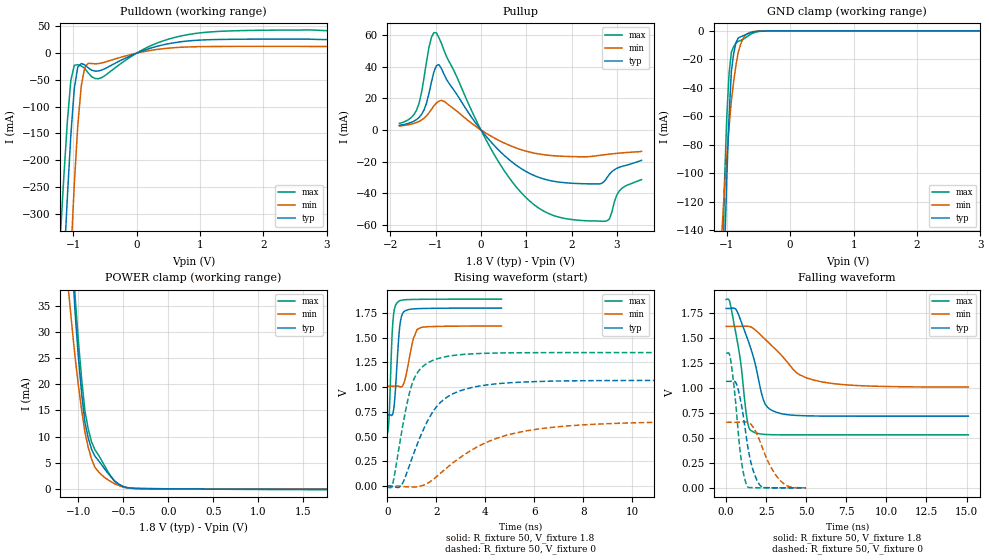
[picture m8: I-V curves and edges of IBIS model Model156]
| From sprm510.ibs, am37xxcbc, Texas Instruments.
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| Model based on original model for DSIPHY_WIO_ADDON_GPIOWRAPPER
|   Sub model FBPB_HS01L10_PU1_1P8
[model]   Model156
|[Input Load]   PU
|[Output Drive] SC01LB10
|Voltage   1.8V
|Mode   I/O
Model_type   I/O
Polarity   Non-Inverting
Enable   Active-Low
Vinl =  0.63
Vinh =  1.17
Cref =  15pF
Rref =  100.0000M
Vref =  0V
Vmeas =  0.9
C_comp   1.429432p   1.270657p   1.602015p
[Model Spec]
Vinl   0.63   0.567   0.6615
Vinh   1.17   1.053   1.2285
[Temperature Range]   25   125   -40
[Voltage Range]   1.8   1.62   1.89
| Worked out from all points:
|   slope of the pulldown table from 0 to 0.27 V, typ, clamps not added: 24.3 ohm
|   slope of the pullup table from 0 to 0.27 V, typ, clamps not added: 29.7 ohm
|   GND clamp passes 1 mA (typ) near -0.60 V on its own axis
|   POWER clamp passes 1 mA (typ) near -0.56 V on its own axis
|   rising waveform, R_fixture 50, V_fixture 1.8: 20-80 % time 175ps typ, 302ps min, 124ps max; typ from 0.72 V to 1.8 V
|   rising waveform, R_fixture 50, V_fixture 0: 20-80 % time 1.3ns typ, 2.85ns min, 687ps max; typ from 0.001 V to 1.07 V
|   falling waveform, R_fixture 50, V_fixture 1.8: 20-80 % time 1.1ns typ, 2.22ns min, 684ps max; typ from 1.8 V to 0.72 V
|   falling waveform, R_fixture 50, V_fixture 0: 20-80 % time 687ps typ, 1.13ns min, 503ps max; typ from 1.07 V to 0.001 V
[POWER_clamp]
-1.8V     362.5mA    191.4mA    412.8mA
-1.109V   56.76mA    37.74mA    60.51mA
-1.073V   44.67mA    31.25mA    47.93mA
-1.036V   33.52mA    25.07mA    36.72mA
-1V       25.06mA    19.75mA    28.2mA
-963.6mV  18.11mA    14.99mA    20.91mA
-927.3mV  12.67mA    10.8mA     14.87mA
-890.9mV  9.734mA    7.935mA    11.44mA
-818.2mV  6.293mA    4.153mA    7.536mA
-636.4mV  2.249mA    1.342mA    2.34mA
-418.2mV  128.7uA    129.3uA    104.4uA
1.764V    -96.73uA   -46.48uA   -163.5uA
[Pulldown]
-1.8V     -1.718A    -2.61A     -1.406A
-1.2V     -527.4mA   -844.5mA   -339.9mA
-1.145V   -396mA     -683.1mA   -229.1mA
-1.091V   -269mA     -526.7mA   -127.5mA
-1.036V   -153.6mA   -378.9mA   -51.17mA
-981.8mV  -66.33mA   -245.6mA   -22.67mA
-927.3mV  -26mA      -136.2mA   -21.54mA
-872.7mV  -19.34mA   -61.98mA   -23.69mA
-763.6mV  -27.2mA    -19.05mA   -36.72mA
-545.5mV  -31.39mA   -18.17mA   -45.46mA
872.7mV   23.46mA    11.88mA    35.92mA
3.545V    25.34mA    12.51mA    41.58mA
[Pullup]
-1.8V     2.903mA    2.423mA    4.112mA
-1.418V   6.595mA    4.711mA    12.64mA
-1.255V   12.69mA    7.42mA     33.24mA
-1.091V   30.4mA     13mA       58.69mA
-981.8mV  40.63mA    17.02mA    61.3mA
-818.2mV  35.38mA    18.12mA    50.59mA
272.7mV   -9.179mA   -4.728mA   -14.55mA
1.255V    -29.75mA   -15.09mA   -48.97mA
2.564V    -34.17mA   -16.31mA   -57.57mA
2.782V    -30.25mA   -15.5mA    -57.49mA
3.055V    -23.63mA   -14.68mA   -38.61mA
3.545V    -19.25mA   -13.56mA   -31.41mA
[GND_clamp]
-1.8V     -2.82A     -1.192A    -3.165A
-1.073V   -235.8mA   -138.4mA   -192.1mA
-1.036V   -159.6mA   -110.8mA   -107.6mA
-1V       -103.8mA   -87.86mA   -60.73mA
-963.6mV  -60.04mA   -67.29mA   -29.86mA
-927.3mV  -28.26mA   -49.09mA   -14.98mA
-890.9mV  -15.95mA   -35.49mA   -11.09mA
-854.5mV  -8.198mA   -24.09mA   -8.559mA
-818.2mV  -4.99mA    -14.87mA   -7.387mA
-709.1mV  -2.858mA   -3.093mA   -5.012mA
-527.3mV  -395.6uA   -260.4uA   -751.2uA
3.6V      0A         0A         0A
[Ramp]
dV/dt_f  0.6499095/1.102807n   0.3669725/2.235766n   0.8166903/0.686518n
dV/dt_r  0.6496235/1.301332n   0.4003589/2.878162n   0.8201376/0.6878106n
R_load = 50
[Rising Waveform]
R_fixture = 50
V_fixture = 1.8
V_fixture_min = 1.62
V_fixture_max = 1.89
0s        719.7mV    1.011V     530.9mV
81ps      721.1mV    1.011V     725.9mV
225ps     731.4mV    1.01V      1.645V
306ps     881.8mV    1.011V     1.804V
387ps     1.19V      1.012V     1.849V
540ps     1.669V     1.003V     1.876V
720ps     1.77V      1.075V     1.884V
1.062ns   1.791V     1.487V     1.887V
1.359ns   1.795V     1.602V     1.888V
4.662ns   1.8V       1.618V     1.89V
[Rising Waveform]
R_fixture = 50
V_fixture = 0
V_fixture_min = 0
V_fixture_max = 0
0s        1.205mV    1.067mV    -8.992mV
225ps     -7.282mV   748.6uV    27.61mV
576ps     10.2mV     -898.2uV   531.9mV
846ps     168.3mV    -6.723mV   879.1mV
1.071ns   324.6mV    -8.466mV   1.072V
1.629ns   651.8mV    27.41mV    1.243V
2.142ns   839.4mV    124.2mV    1.295V
4.041ns   1.023V     441.9mV    1.343V
6.246ns   1.058V     581mV      1.349V
19.67ns   1.069V     657.1mV    1.35V
[Falling Waveform]
R_fixture = 50
V_fixture = 1.8
V_fixture_min = 1.62
V_fixture_max = 1.89
0s        1.8V       1.62V      1.89V
297ps     1.801V     1.62V      1.812V
846ps     1.707V     1.62V      1.325V
1.296ns   1.51V      1.622V     696.5mV
1.602ns   1.365V     1.609V     570.6mV
2.331ns   879mV      1.506V     538.4mV
3.285ns   751.5mV    1.358V     533.2mV
4.473ns   726.8mV    1.147V     532.6mV
5.904ns   721.2mV    1.066V     532.6mV
15.11ns   720mV      1.012V     532.6mV
[Falling Waveform]
R_fixture = 50
V_fixture = 0
V_fixture_min = 0
V_fixture_max = 0
0s        1.069V     658.7mV    1.35V
279ps     1.07V      658.9mV    1.283V
666ps     1.033V     658.8mV    721.8mV
972ps     814.5mV    661.6mV    244.7mV
1.305ns   458.1mV    660.3mV    20.53mV
1.674ns   181.1mV    612.8mV    3.333mV
2.187ns   15.44mV    435.5mV    1.951mV
2.772ns   2.813mV    213.9mV    1.792mV
3.465ns   1.692mV    61.59mV    1.775mV
4.968ns   1.433mV    2.606mV    1.773mV
